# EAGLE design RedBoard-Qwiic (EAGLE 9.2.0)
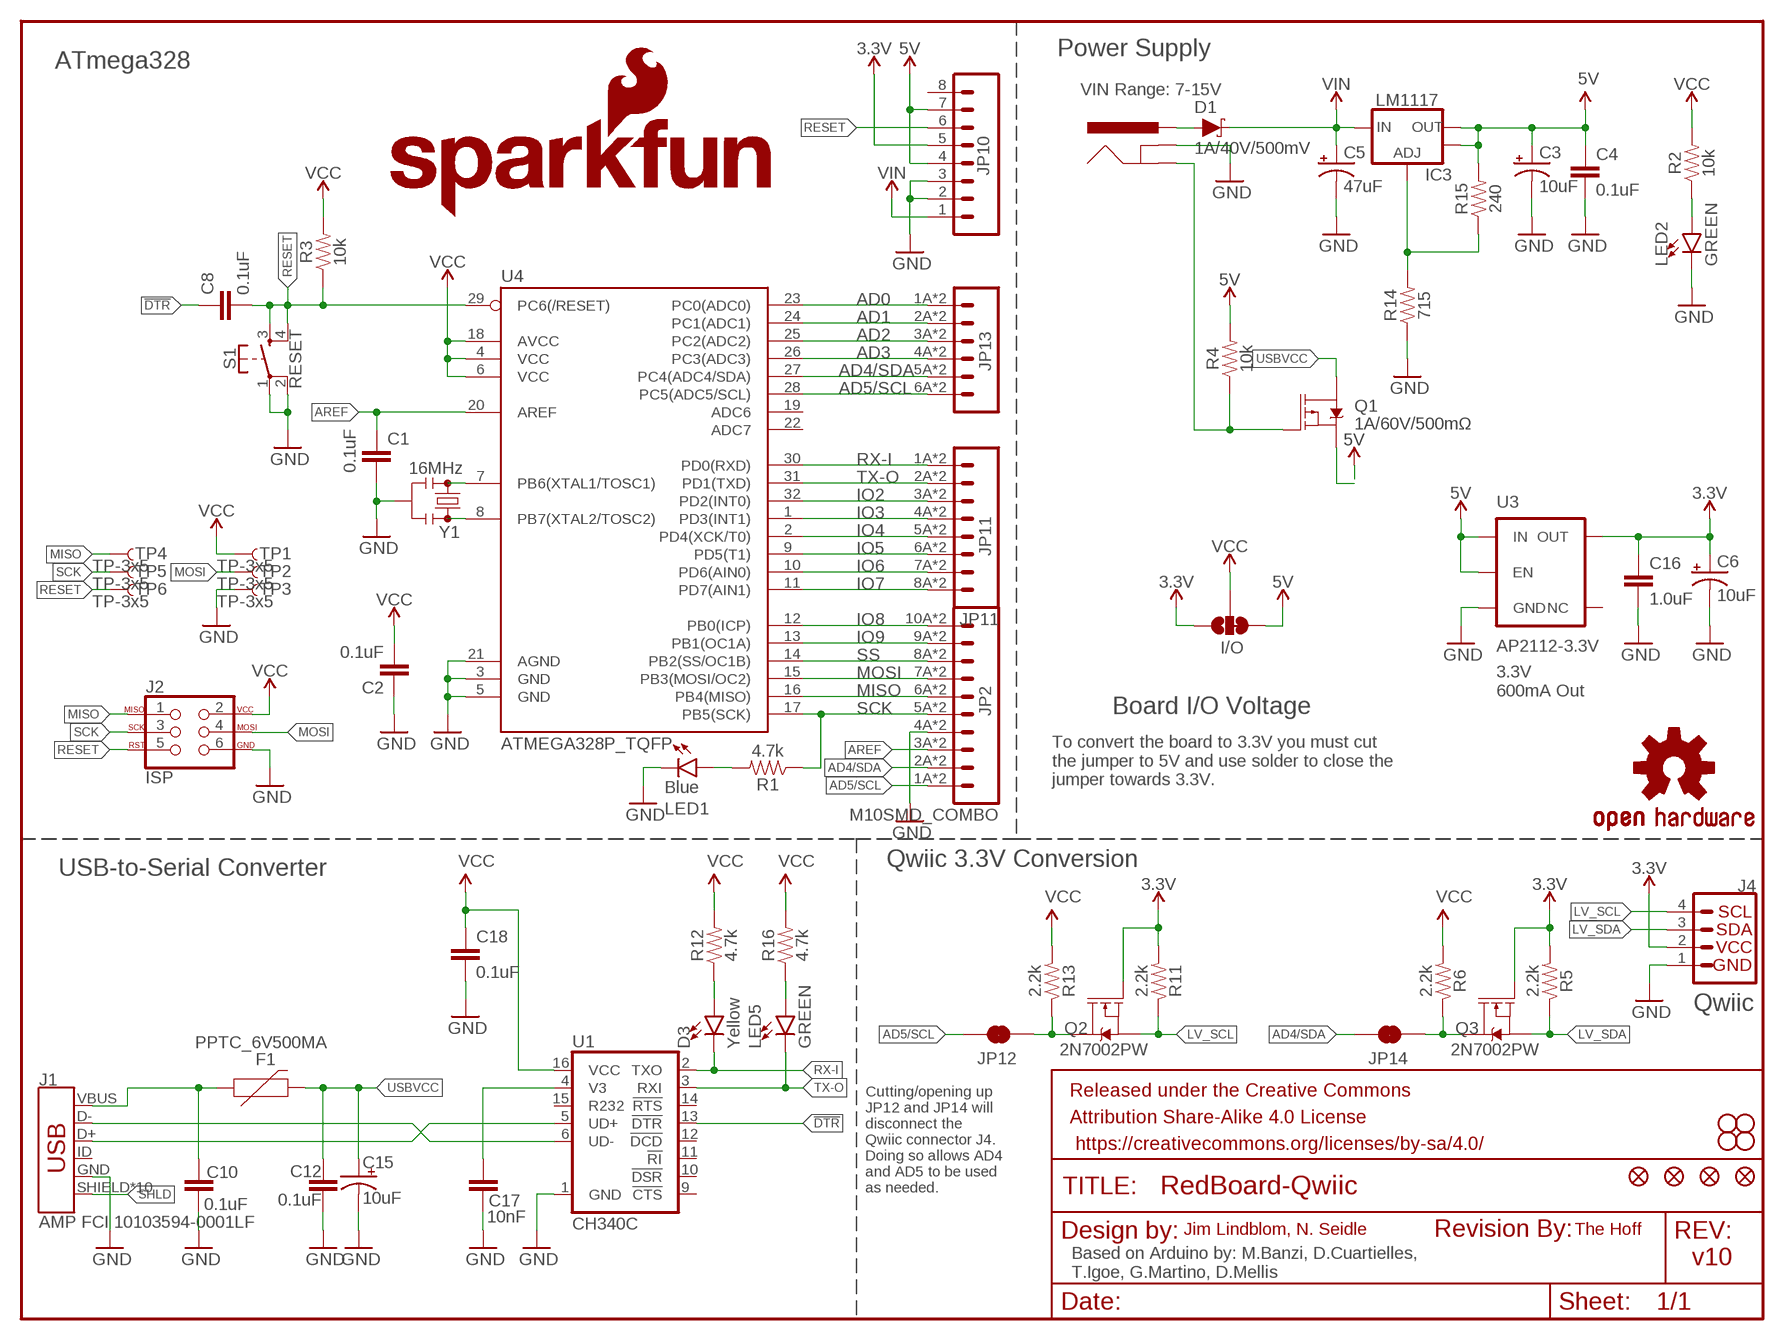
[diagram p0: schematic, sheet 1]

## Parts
C1  0.1uF  0.1UF-0603-25V-(+80/-20%)  [0603]
C2  0.1uF  0.1UF-0603-25V-(+80/-20%)  [0603]
C3  10uF  10UF-POLAR-EIA3216-16V-10%(TANT)  [EIA3216]
C4  0.1uF  0.1UF-0603-25V-(+80/-20%)  [0603]
C5  47uF  47UF-POLAR-PANASONIC_D-35V-20%  [PANASONIC_D]
C6  10uF  10UF-POLAR-EIA3216-16V-10%(TANT)  [EIA3216]
C8  0.1uF  0.1UF-0603-25V-(+80/-20%)  [0603]
C10  0.1uF  0.1UF-0603-25V-(+80/-20%)  [0603]
C12  0.1uF  0.1UF-0603-25V-(+80/-20%)  [0603]
C15  10uF  10UF-POLAR-EIA3216-16V-10%(TANT)  [EIA3216]
C16  1.0uF  1.0UF-16V-10%(0603)  [0603-CAP]
C17  10nF  10NF/10000PF-50V-10%(0603)  [0603-CAP]
C18  0.1uF  0.1UF-0603-25V-(+80/-20%)  [0603]
D1  1A/40V/500mV  DIODE-SCHOTTKY-SS14  [SMA-DIODE]
D3  Yellow  LED-YELLOW_HIDDENSILK  [LED-1206-HIDDENSILK]
F1  PPTC_6V500MA  [0805]
FRAME2  FRAME-LETTER  [CREATIVE_COMMONS]
I/O  JUMPER-SMT_3_1-NC_TRACE_SILK  [SMT-JUMPER_3_1-NC_TRACE_SILK]
IC3  LM1117  V_REG_LM1117ALT1  [SOT223-ALT1]
J1  AMP FCI 10103594-0001LF  USB_MICRO-B_HALF_PTH_MILL  [USB-MICROB-PTH-MILL]
J2  ISP  AVR_SPI_PROG_3X2SMD  [2X3_SMT_POSTS]
J3  POWER_JACKSUPER_BOMB_DIGITY  [POWER_JACK_SMD_OVERPASTE_SUPER_BOMB_DIGITY]
J4  QWIIC_CONNECTORJS-1MM  [1X04_1MM_RA]
JP1  SFE_LOGO_NAME.1_INCH  [SFE_LOGO_NAME_.1]
JP2  M10SMD_COMBO  [1X10_SMD_COMBINED]
JP3  STAND-OFF  [STAND-OFF]
JP4  STAND-OFF  [STAND-OFF]
JP5  STAND-OFF  [STAND-OFF]
JP6  STAND-OFF  [STAND-OFF]
JP7  SFE_LOGO_FLAME.1_INCH  [SFE_LOGO_FLAME_.1]
JP8  FIDUCIAL1X2  [FIDUCIAL-1X2]
JP9  FIDUCIAL1X2  [FIDUCIAL-1X2]
JP10  CONN_08SMD-COMBO-FEMALE  [1X08_SMD_COMBINED]
JP11  JP11  M08SMD-COMBO  [1X08_SMD_COMBINED@1]
JP12  JUMPER-SMT_2_NC_TRACE_SILK  [SMT-JUMPER_2_NC_TRACE_SILK]
JP13  M06SMD-STRAIGHT-COMBO  [1X06_SMD_STRAIGHT_COMBO]
JP14  JUMPER-SMT_2_NC_TRACE_SILK  [SMT-JUMPER_2_NC_TRACE_SILK]
JP15  FIDUCIAL1X2  [FIDUCIAL-1X2]
JP16  FIDUCIAL1X2  [FIDUCIAL-1X2]
LED1  Blue  LED-BLUE_HIDDENSILK  [LED-1206-HIDDENSILK]
LED2  GREEN  LED-GREEN_HIDDENSILK  [LED-1206-HIDDENSILK]
LED5  GREEN  LED-GREEN_HIDDENSILK  [LED-1206-HIDDENSILK]
LOGO1  REVISION  [REVISION]
Q1  1A/60V/500mΩ  MOSFET-PCH-ZXMP6A13F  [SOT23-3]
Q2  2N7002PW  MOSFET-NCH-2N7002PW  [SOT323]
Q3  2N7002PW  MOSFET-NCH-2N7002PW  [SOT323]
R1  4.7k  4.7KOHM-0603-1/10W-1%  [0603]
R2  10k  10KOHM-0603-1/10W-1%  [0603]
R3  10k  10KOHM-0603-1/10W-1%  [0603]
R4  10k  10KOHM-0603-1/10W-1%  [0603]
R5  2.2k  2.2KOHM-0603-1/10W-1%  [0603]
R6  2.2k  2.2KOHM-0603-1/10W-1%  [0603]
R11  2.2k  2.2KOHM-0603-1/10W-1%  [0603]
R12  4.7k  4.7KOHM-0603-1/10W-1%  [0603]
R13  2.2k  2.2KOHM-0603-1/10W-1%  [0603]
R14  715  715OHM-0603-1/10W-1%  [0603]
R15  240  240OHM-0603-1/10W-1%  [0603]
R16  4.7k  4.7KOHM-0603-1/10W-1%  [0603]
S1  RESET  MOMENTARY-SWITCH-SPST-2-SMD-5.2MM-TALL  [TACTILE_SWITCH_SMD_5.2MM]
TP1  TP-3x5  TEST-POINT3X5  [PAD.03X.05]
TP2  TP-3x5  TEST-POINT3X5  [PAD.03X.05]
TP3  TP-3x5  TEST-POINT3X5  [PAD.03X.05]
TP4  TP-3x5  TEST-POINT3X5  [PAD.03X.05]
TP5  TP-3x5  TEST-POINT3X5  [PAD.03X.05]
TP6  TP-3x5  TEST-POINT3X5  [PAD.03X.05]
U1  CH340C  [SO016]
U3  AP2112-3.3V  V_REG_AP2112K-3.3V  [SOT23-5]
U4  ATMEGA328P_TQFP  [TQFP32-08]
U$16  OSHW-LOGOS  [OSHW-LOGO-S]
Y1  16MHz  RESONATOR-16MHZSMD_3.2X1.3  [RESONATOR-SMD-3.2X1.3]

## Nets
3.3V: C6.+ C16.1 I/O.1 J4.2 JP10.5 Q2.1(G) Q3.1(G) R5.2 R11.2 U3.5(OUT)
5V: C3.+ C4.1 I/O.3 IC3.2(OUT) IC3.4(OUT) JP10.4 JP10.7 Q1.2(S) R4.2 R15.2 U3.1(IN) U3.3(EN)
!DTR: C8.1 U1.13(!DTR)
AD0: JP13.1A JP13.1B U4.23(PC0(ADC0))
AD1: JP13.2A JP13.2B U4.24(PC1(ADC1))
AD2: JP13.3A JP13.3B U4.25(PC2(ADC2))
AD3: JP13.4A JP13.4B U4.26(PC3(ADC3))
AD4/SDA: JP2.2A JP2.2B JP13.5A JP13.5B JP14.2 U4.27(PC4(ADC4/SDA))
AD5/SCL: JP2.1A JP2.1B JP12.2 JP13.6A JP13.6B U4.28(PC5(ADC5/SCL))
AREF: C1.1 JP2.3A JP2.3B U4.20(AREF)
GND: C1.2 C2.1 C3.- C4.2 C5.- C6.- C10.2 C12.2 C15.- C16.2 C17.2 C18.2 J1.GND J2.6 J3.GND(GNDBREAK) J4.1 JP2.4A JP2.4B JP10.2 JP10.3 LED1.C LED2.C R14.1 S1.1 S1.2 TP3.P$1 U1.1(GND) U3.2(GND) U4.3(GND) U4.5(GND) U4.21(AGND) Y1.2
INSERT: J3.P$4(GND) Q1.1(G) R4.1
IO2: JP11.3A JP11.3B U4.32(PD2(INT0))
IO3: JP11.4A JP11.4B U4.1(PD3(INT1))
IO4: JP11.5A JP11.5B U4.2(PD4(XCK/T0))
IO5: JP11.6A JP11.6B U4.9(PD5(T1))
IO6: JP11.7A JP11.7B U4.10(PD6(AIN0))
IO7: JP11.8A JP11.8B U4.11(PD7(AIN1))
IO8: JP2.10A JP2.10B U4.12(PB0(ICP))
IO9: JP2.9A JP2.9B U4.13(PB1(OC1A))
LV_SCL: J4.4 Q2.2(S) R11.1
LV_SDA: J4.3 Q3.2(S) R5.1
MISO: J2.1 JP2.6A JP2.6B TP4.P$1 U4.16(PB4(MISO))
MOSI: J2.4 JP2.7A JP2.7B TP2.P$1 U4.15(PB3(MOSI/OC2))
N$1: LED1.A R1.2
N$2: LED2.A R2.1
N$3: U4.7(PB6(XTAL1/TOSC1)) Y1.1
N$4: U4.8(PB7(XTAL2/TOSC2)) Y1.3
N$5: LED5.A R16.1
N$6: C17.1 U1.4(V3)
N$7: JP12.1 Q2.3(D) R13.1
N$8: JP14.1 Q3.3(D) R6.1
N$9: D3.A R12.1
N$13: J1.D- U1.6(UD-)
N$14: J1.D+ U1.5(UD+)
N$15: IC3.1(ADJ) R14.2 R15.1
PWRIN: D1.A J3.VIN0(PWR)
RESET: C8.2 J2.5 JP10.6 R3.1 S1.3 S1.4 TP6.P$1 U4.29(PC6(/RESET))
RX-I: D3.C JP11.1A JP11.1B U1.2(TXO) U4.30(PD0(RXD))
SCK: J2.3 JP2.5A JP2.5B R1.1 TP5.P$1 U4.17(PB5(SCK))
SHLD: J1.SHIELD J1.SHIELD2(SHIELD) J1.SHIELD3(SHIELD) J1.SHIELD4(SHIELD) J1.SHIELD5(SHIELD) J1.SHIELD6(SHIELD) J1.SHIELD7(SHIELD) J1.SHIELD8(SHIELD) J1.SHIELD9(SHIELD) J1.SHIELD10(SHIELD)
SS: JP2.8A JP2.8B U4.14(PB2(SS/OC1B))
TX-O: JP11.2A JP11.2B LED5.C U1.3(RXI) U4.31(PD1(TXD))
USBVCC: C12.1 C15.+ F1.2 Q1.3(D)
VCC: C2.2 C18.1 I/O.2 J2.2 R2.2 R3.2 R6.2 R12.2 R13.2 R16.2 TP1.P$1 U1.16(VCC) U4.4(VCC) U4.6(VCC) U4.18(AVCC)
VIN: C5.+ D1.C IC3.3(IN) JP10.1
VUSB: C10.1 F1.1 J1.VBUS
Unconnected: J1.ID JP10.8 U1.9(!CTS) U1.10(!DSR) U1.11(!RI) U1.12(!DCD) U1.14(!RTS) U1.15(R232) U3.4(NC) U4.19(ADC6) U4.22(ADC7)

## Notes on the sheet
- Power Supply
- ATmega328
- VIN Range: 7-15V
- 3.3V
  600mA Out
- Board I/O Voltage
- To convert the board to 3.3V you must cut
  the jumper to 5V and use solder to close the
  jumper towards 3.3V.
- Qwiic 3.3V Conversion
- USB-to-Serial Converter
- Qwiic
- Cutting/opening up
  JP12 and JP14 will 
  disconnect the 
  Qwiic connector J4.  
  Doing so allows AD4 
  and AD5 to be used
  as needed.
- Jim Lindblom, N. Seidle | The Hoff
- v10
- Based on Arduino by: M.Banzi, D.Cuartielles, 
  T.Igoe, G.Martino, D.Mellis

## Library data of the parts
C1 C2 C4 C8 C10 C12 C18 = SparkFun-Capacitors:0.1UF: 0.1µF ceramic capacitors; PROD_ID: CAP-00810
C3 C6 C15 = SparkFun-Capacitors:10UF-POLAR: 10.0µF polarized capacitors; PROD_ID: CAP-00811
C5 = SparkFun-Capacitors:47UF-POLAR: 47µF polarized capacitors; PROD_ID: CAP-08478
C16 = SparkFun-Capacitors:1.0UF-16V-10%(0603): CAP-00868; PROD_ID: CAP-00868
C17 = SparkFun-Capacitors:10NF/10000PF-50V-10%(0603): CAP-00867; PROD_ID: CAP-00867
D1 = SparkFun-DiscreteSemi:DIODE-SCHOTTKY: Schottky diode; PROD_ID: DIO-08053
D3 = SparkFun-LED:LED-YELLOW: Yellow SMD LED; PROD_ID: DIO-09909
F1 = SparkFun-Fuses:PPTC: Resettable Fuse PPTC
FRAME2 = SparkFun-Aesthetics:FRAME-LETTER: Schematic Frame - Letter
I/O = SparkFun-Jumpers:JUMPER-SMT_3_1-NC_TRACE: Normally closed trace jumper (1 of 2 connections) This jumper has a trace between two pads so it's normally closed (NC). The other connection is normally open (NO). Use a razor knife to open the connection. For best results follow the IPC guidelines for cutting traces: Cutout at least 0.063 mm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
IC3 = Testing:V_REG_LM1117: Voltage Regulator LM1117 Standard adjustable voltage regulator but in SMD form. Spark Fun Electronics SKU : COM-00595; PROD_ID: VREG-08170
J1 = SparkFun-Connectors:USB_MICRO-B: USB Type Micro-B Connector Male/female and PTH/SMT variants SparkFun Products: SparkFun microB USB Breakout SparkFun USB microB Plug Breakout SparkFun ESP8266 Thing; PROD_ID: CONN-13711
J2 = SparkFun-Connectors:AVR_SPI_PROG_3X2: AVR ISP 6 Pin This is the reduced ISP connector for AVR programming. Common on Arduino. This footprint will take up less PCB space and can be used with a 10-pin to 6-pin adapter such as SKU: BOB-08508 **Special note about "TEST_POINT" package. The stop mask is on the top side, so if you want your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; PROD_ID: CONN-11415
J3 = Testing:POWER_JACK: Power Jack This is the standard 5.5mm barrel jack for power. The PTH is the most common, proven, reliable, footprint. All others are experimental. The Slot footprint only works if the mill layer is transmitted to the PCB fab house so be warned. Spark Fun Electronics SKU : PRT-00119. Mating wall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; PROD_ID: CONN-08106
J4 = SparkFun-Connectors:QWIIC_CONNECTOR: SparkFun I2C Standard Qwiic Connector An SMD 1mm pitch JST connector makes it easy and quick (get it? Qwiic?) to connect I2C devices to each other. The Qwiic system enables fast and solderless connection between popular platforms and various sensors and actuators. We carry 200mm, 100mm, 50mm, and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; PROD_ID: CONN-13694
JP1 = SparkFun-Aesthetics:SFE_LOGO_NAME: SFE Logo, name only
JP2 = SparkFun-Connectors:M10: Header 10 Standard 10-pin 0.1" header. Use with straight break away headers (SKU : PRT-00116), right angle break away headers (PRT-00553), swiss pins (PRT-00743), machine pins (PRT-00117), and female headers (PRT-00115).; PROD_ID: CONN-11219
JP3-JP6 = SparkFun:STAND-OFF: Stand Off
JP7 = SparkFun-Aesthetics:SFE_LOGO_FLAME: SFE Logo, flame only
JP8 JP9 JP15 JP16 = SparkFun:FIDUCIAL: Fiducial Alignment Points
JP10 = SparkFun-Connectors:CONN_08: Multi connection point. Often used as Generic Header-pin footprint for 0.1 inch spaced/style header connections On any of the 0.1 inch spaced packages, you can populate with these: Break Away Headers - Straight (PRT-00116) Break Away Male Headers - Right Angle (PRT-00553) Female Headers (PRT-00115)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; PROD_ID: CONN-10204; SF_ID: PRT-11543
JP11 = SparkFun-Connectors:M08: Header 8 Standard 8-pin 0.1" header. Use with straight break away headers (SKU : PRT-00116), right angle break away headers (PRT-00553), swiss pins (PRT-00743), machine pins (PRT-00117), and female headers (PRT-00115).; PROD_ID: CONN-10204
JP12 JP14 = SparkFun-Jumpers:JUMPER-SMT_2_NC_TRACE: Normally closed trace jumper
JP13 = SparkFun-Connectors:M06: Header 6 Standard 6-pin 0.1" header. Use with straight break away headers (SKU : PRT-00116), right angle break away headers (PRT-00553), swiss pins (PRT-00743), machine pins (PRT-00117), and female headers (PRT-00115). Molex polarized connector foot print use with SKU : PRT-08094 with associated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; PROD_ID: CONN-10203
LED1 = SparkFun-LED:LED-BLUE: Blue SMD LED; PROD_ID: DIO-09911
LED2 = SparkFun-LED:LED-GREEN: Green SMD LED; PROD_ID: DIO-09910
LED5 = SparkFun-LED:LED-GREEN: Green SMD LED; PROD_ID: DIO-00862
LOGO1 = SparkFun-Aesthetics:REVISION: "Revision By" Text
Q1 = SparkFun-DiscreteSemi:MOSFET-PCH: P-channel MOSFETs Voltage controlled devices that allow control of high current outputs.; PROD_ID: TRANS-08285
Q2 Q3 = SparkFun-DiscreteSemi:MOSFET-NCH: N-channel MOSFETs Voltage controlled devices that allow control of high current outputs.; PROD_ID: TRANS-11151; VALUE: 310mA/60V/1.6Ω
R1 R12 R16 = SparkFun-Resistors:4.7KOHM: 4.7kΩ resistor; PROD_ID: RES-07857
R2-R4 = SparkFun-Resistors:10KOHM: 10kΩ resistor; PROD_ID: RES-00824
R5 R6 R11 R13 = SparkFun-Resistors:2.2KOHM: 2.2kΩ resistor; PROD_ID: RES-08272
R14 = SparkFun-Resistors:715OHM: 715Ω resistor; PROD_ID: RES-07850
R15 = SparkFun-Resistors:240OHM: 240Ω resistor; PROD_ID: RES-07849
S1 = SparkFun-Switches:MOMENTARY-SWITCH-SPST-2: Momentary Switch (Pushbutton) - SPST - Two Circuits Normally-open (NO) SPST momentary switches (buttons, pushbuttons). Schematic symbol includes two switch circuits. Variants SMD-4.6MMX2.8MM - 4.60mm x 2.80mm Tactile Momentary Button Switch - Used on SparkFun SAMD21 Mini Breakout SMD-5.2MM - Mini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; PROD_ID: SWCH-14139
TP1-TP4 TP6 = SparkFun-Connectors:TEST-POINT: Bare copper test points for troubleshooting or ICT
TP5 = SparkFun-Passives:TEST-POINT: Bare copper test points for troubleshooting or ICT
U1 = SparkFun-IC-Comms:CH340C; PROD_ID: IC-14038
U3 = SparkFun-PowerIC:V_REG_AP2112: AP2112 - 600mA CMOS LDO Regulator w/ Enable The AP2112 is CMOS process low dropout linear regulator with enable function, the regulator delivers a guaranteed 600mA (min.) continuous load current. Features Output Voltage Accuracy: ±1.5% Output Current: 600mA (Min.) Foldback Short Current Protection: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; PROD_ID: VREG-12457; VALUE: 3.3V
U4 = SparkFun-IC-Microcontroller:ATMEGA328P_TQFP; PROD_ID: IC-09069
U$16 = SparkFun-Aesthetics:OSHW-LOGO: Open Source Hardware Logo
Y1 = SparkFun-Clocks:RESONATOR-16MHZ: 16MHz Resonator Digikey Example Frequency: 16MHz Frequency Stability: &plusmn;0.3% Frequency Tolerance: &plusmn;0.5% Capacitance: 15pF; PROD_ID: XTAL-08900

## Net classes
1 power: width 0.178 mm

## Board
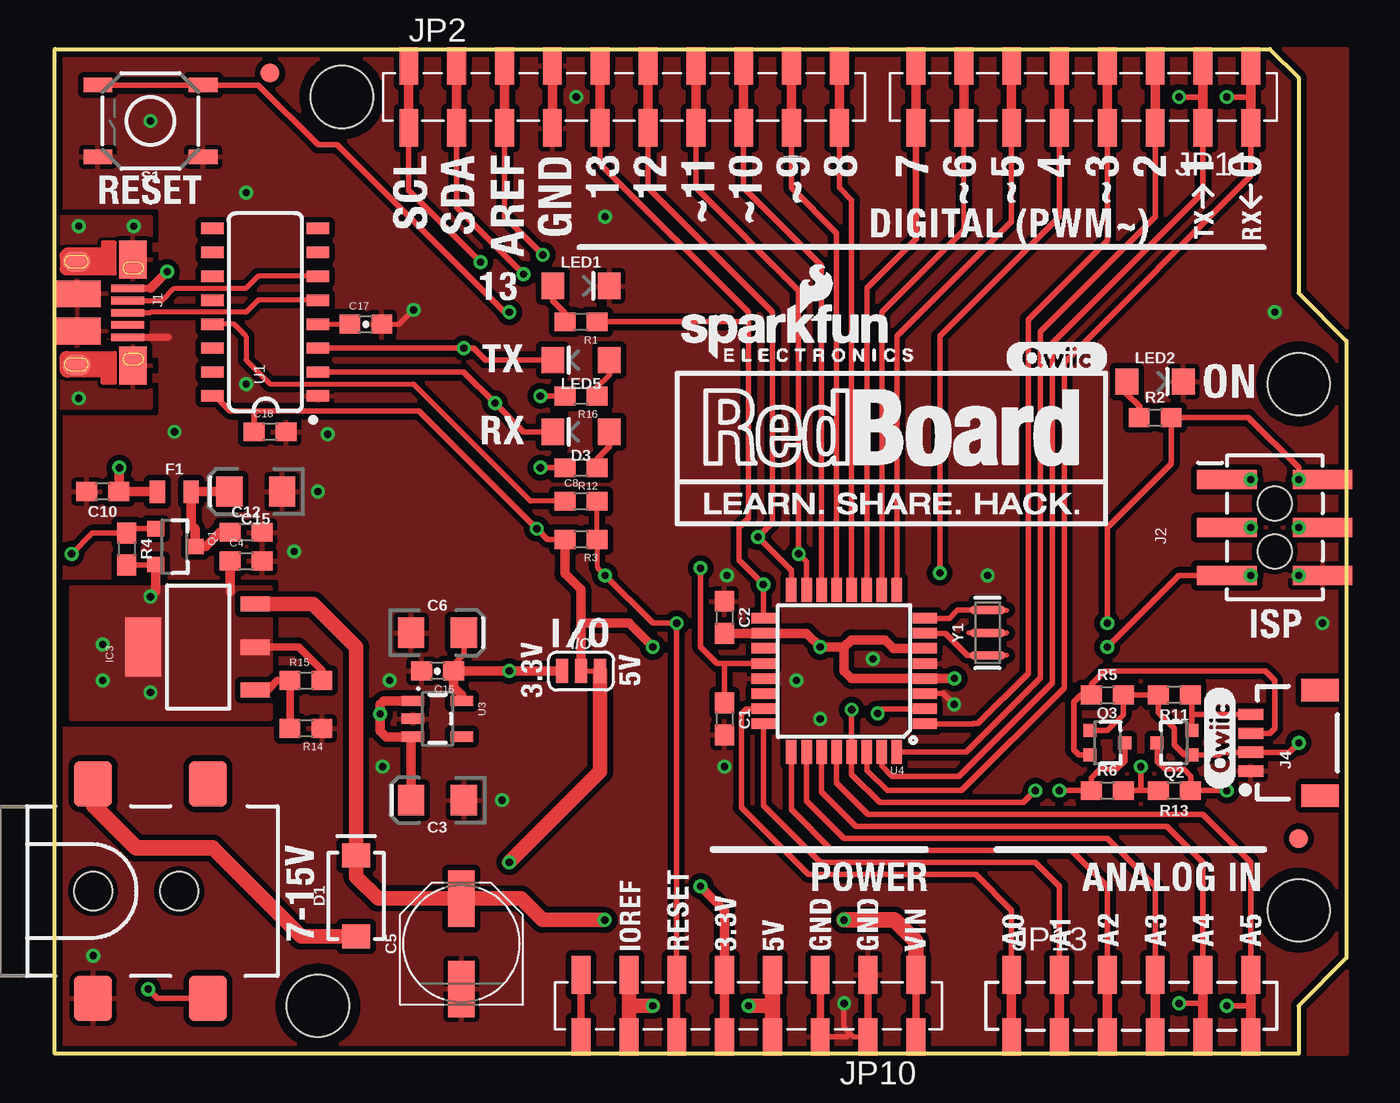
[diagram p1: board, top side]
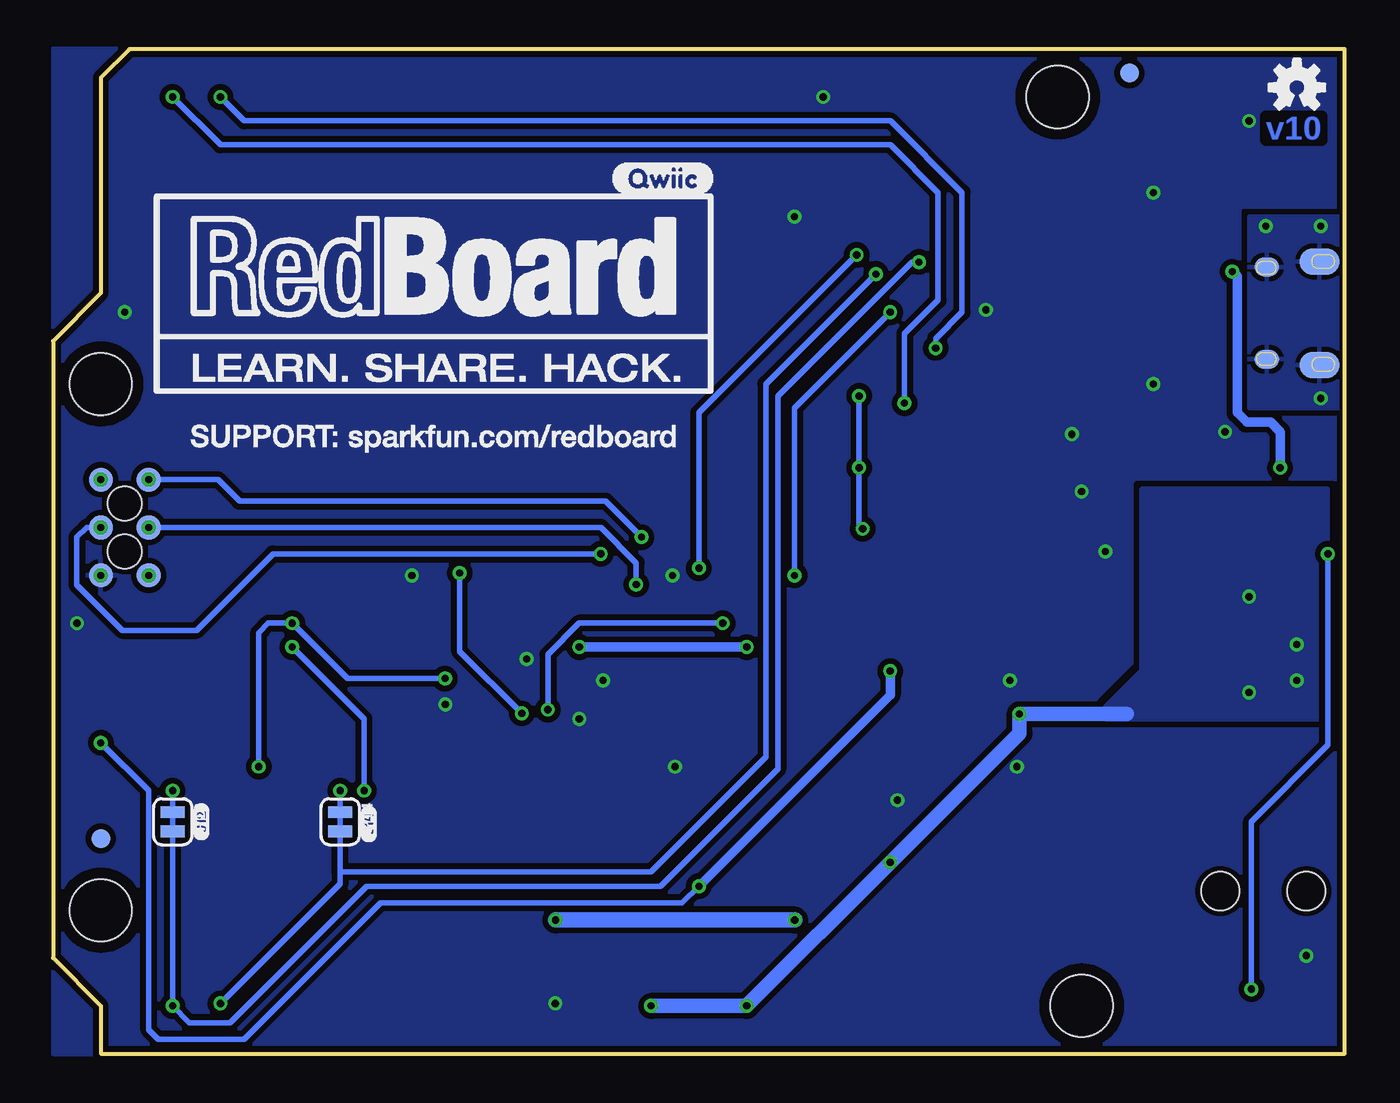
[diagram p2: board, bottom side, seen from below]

Size 68.58 x 53.34 mm. Coordinates in mm from the lower left corner, seen from the top.
Outline: 0,53.34 64.52,53.34 66.04,51.82 66.04,40.39 68.58,37.85 68.58,5.08 66.04,2.54 66.04,0 0,0 0,53.34
Copper layers (1*16): Top 0.035mm / dielectric 1.5mm / Bottom 0.035mm
Design rules "SparkFun-2-layer-TIGHT": minimum track width 7mil, minimum drill 15mil, track to track 7mil, track to pad 7mil, pad to pad 7mil, via to via 7mil, smd to smd 7mil, copper to edge 7mil, drill to drill 7mil, minimum pad ring 7mil, minimum via ring 7mil, stop-mask expansion 4mil, vias tented up to drill 25mil, thermal gap 10mil
vRestrict: area 0.6,22.4 to 2,30.6; area 5.7,23.1 to 7.4,30.6; area 47.9,10.8 to 48.5,11.3; area 50.4,10.7 to 50.9,11.6; area 11.3,29.3 to 12.7,31.6; area 0.3,13 to 9.4,25

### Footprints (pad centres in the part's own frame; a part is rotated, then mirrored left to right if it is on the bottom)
0603 = smd 1.1 x 1: 1 -0.85,0; 2 0.85,0
EIA3216 = smd 1.4 x 1.6: + 1.4,0; - -1.4,0
PANASONIC_D = smd 3 x 1.4: + 2.4,0; - -2.4,0
0603-CAP = smd 1.1 x 1: 1 -0.85,0; 2 0.85,0
SMA-DIODE = smd 1.27 x 1.47: A -2.15,0; C 2.15,0
LED-1206-HIDDENSILK = smd 1.2 x 1.4: A -1.5,0; C 1.5,0
0805 = smd 0.8 x 1.2: 1 -0.9,0; 2 0.9,0
SMT-JUMPER_3_1-NC_TRACE_SILK = smd 0.635 x 1.27: 1 -1.016,0; 2 0,0; 3 1.016,0
SOT223-ALT1 = smd 0.813 x 1.524: 1 -2.271,-3.02; 2 0,-3.02; 3 2.288,-3.02 | smd 3.124 x 1.905: 4 0,2.921
USB-MICROB-PTH-MILL = smd 0.4 x 1.75: D+ 0.031,1.331; D- -0.619,1.331; GND 1.331,1.331; ID 0.681,1.331; VBUS -1.269,1.331 | smd 2 x 1.46: SHIELD -2.794,1.606; SHIELD2 2.831,1.606 | smd 1.425 x 2.5: SHIELD3 -0.979,-1.349; SHIELD4 0.996,-1.352 | smd 1.4 x 2.1 bottom: SHIELD5 -2.7,-1.2; SHIELD7 2.8,-1.2 | smd 1.1 x 1.5: SHIELD6 2.8,-1.4; SHIELD8 -2.7,-1.4 | smd 1 x 1.3 bottom: SHIELD9 -2.4,1.6; SHIELD10 2.5,1.6
2X3_SMT_POSTS = smd 1 x 3.17: 1 -2.54,-2.54; 2 -2.54,2.54; 3 0,-2.54; 4 0,2.54; 5 2.54,-2.54; 6 2.54,2.54 | hole 1.8: -1.27,0; 1.27,0
POWER_JACK_SMD_OVERPASTE_SUPER_BOMB_DIGITY = smd 2 x 2.4: GND 0,-5.7; P$4 6.1,-5.7; VIN0 0,5.7; VIN1 6.1,5.7 | hole 2.032: 0,0; 4.572,0
1X04_1MM_RA = smd 0.6 x 1.35: 1 -1.5,0; 2 -0.5,0; 3 0.5,0; 4 1.5,0 | smd 1.2 x 2: NC1 2.8,-3.675; NC2 -2.8,-3.675
1X10_SMD_COMBINED = smd 1 x 2: 1A 0,1.65; 1B 0,-1.65; 2A 2.54,1.65; 2B 2.54,-1.65; 3A 5.08,1.65; 3B 5.08,-1.65; 4A 7.62,1.65; 4B 7.62,-1.65; 5A 10.16,1.65; 5B 10.16,-1.65; 6A 12.7,1.65; 6B 12.7,-1.65; 7A 15.24,1.65; 7B 15.24,-1.65; 8A 17.78,1.65; 8B 17.78,-1.65; 9A 20.32,1.65; 9B 20.32,-1.65; 10A 22.86,1.65; 10B 22.86,-1.65
STAND-OFF = hole 3.302: 0,0
FIDUCIAL-1X2 = smd 1 x 1: 1 0,0
1X08_SMD_COMBINED = smd 1 x 2: 1 0,1.65; 1@2 0,-1.65; 2 2.54,-1.65; 2@2 2.54,1.65; 3 5.08,1.65; 3@2 5.08,-1.65; 4 7.62,-1.65; 4@2 7.62,1.65; 5 10.16,1.65; 5@2 10.16,-1.65; 6 12.7,-1.65; 6@2 12.7,1.65; 7 15.24,1.65; 7@2 15.24,-1.65; 8 17.78,-1.65; 8@2 17.78,1.65
1X08_SMD_COMBINED@1 = smd 1 x 2: 1A 0,1.65; 1B 0,-1.65; 2A 2.54,-1.65; 2B 2.54,1.65; 3A 5.08,1.65; 3B 5.08,-1.65; 4A 7.62,-1.65; 4B 7.62,1.65; 5A 10.16,1.65; 5B 10.16,-1.65; 6A 12.7,-1.65; 6B 12.7,1.65; 7A 15.24,1.65; 7B 15.24,-1.65; 8A 17.78,-1.65; 8B 17.78,1.65
SMT-JUMPER_2_NC_TRACE_SILK = smd 0.635 x 1.27: 1 -0.508,0; 2 0.508,0
1X06_SMD_STRAIGHT_COMBO = smd 1 x 2: 1A 0,-1.65; 1B 0,1.65; 2A 2.54,1.65; 2B 2.54,-1.65; 3A 5.08,-1.65; 3B 5.08,1.65; 4A 7.62,1.65; 4B 7.62,-1.65; 5A 10.16,-1.65; 5B 10.16,1.65; 6A 12.7,1.65; 6B 12.7,-1.65
SOT23-3 = smd 0.8 x 0.9: 1 -0.95,-1; 2 0.95,-1; 3 0,1.1
SOT323 = smd 0.7 x 0.7: 1 -0.65,-0.925; 2 0.65,-0.925; 3 0,0.925
TACTILE_SWITCH_SMD_5.2MM = smd 1.524 x 0.762: 1 -2.794,1.905; 2 2.794,1.905; 3 -2.794,-1.905; 4 2.794,-1.905
PAD.03X.05 = smd 1.27 x 1.27: P$1 0,0
SO016 = smd 0.6 x 1.2: 1 -4.445,-2.8; 2 -3.175,-2.8; 3 -1.905,-2.8; 4 -0.635,-2.8; 5 0.635,-2.8; 6 1.905,-2.8; 7 3.175,-2.8; 8 4.445,-2.8; 9 4.445,2.8; 10 3.175,2.8; 11 1.905,2.8; 12 0.635,2.8; 13 -0.635,2.8; 14 -1.905,2.8; 15 -3.175,2.8; 16 -4.445,2.8
SOT23-5 = smd 0.55 x 1.2: 1 -0.95,-1.3; 2 0,-1.3; 3 0.95,-1.3; 4 0.95,1.3; 5 -0.95,1.3
TQFP32-08 = smd 1.27 x 0.559: 1 -4.293,2.8; 2 -4.293,2; 3 -4.293,1.2; 4 -4.293,0.4; 5 -4.293,-0.4; 6 -4.293,-1.2; 7 -4.293,-2; 8 -4.293,-2.8; 17 4.293,-2.8; 18 4.293,-2; 19 4.293,-1.2; 20 4.293,-0.4; 21 4.293,0.4; 22 4.293,1.2; 23 4.293,2; 24 4.293,2.8 | smd 0.559 x 1.27: 9 -2.8,-4.293; 10 -2,-4.293; 11 -1.2,-4.293; 12 -0.4,-4.293; 13 0.4,-4.293; 14 1.2,-4.293; 15 2,-4.293; 16 2.8,-4.293; 25 2.8,4.293; 26 2,4.293; 27 1.2,4.293; 28 0.4,4.293; 29 -0.4,4.293; 30 -1.2,4.293; 31 -2,4.293; 32 -2.8,4.293
RESONATOR-SMD-3.2X1.3 = smd 0.45 x 1.905: 1 -1.2,0; 2 0,0; 3 1.2,0

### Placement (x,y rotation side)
C1  35.56,17.78 270 top
C2  35.56,23.17 270 top
C3  20.32,13.46 180 top
C4  10.16,26.16 0 top
C5  21.59,5.84 90 top
C6  20.32,22.35 0 top
C8  27.94,29.34 0 top
C10  2.54,29.84 180 top
C12  10.16,27.69 0 top
C15  10.67,29.84 180 top
C16  20.32,20.32 180 top
C17  16.51,38.73 0 top
C18  11.43,33.02 0 top
D1  16,8.38 90 top
D3  27.94,33.02 180 top
F1  6.35,29.84 0 top
FRAME2  not placed on the board
I/O  27.94,20.32 0 top
IC3  7.62,21.59 90 top
J1  2.54,39.37 270 top
J2  64.77,27.94 270 top
J3  2.03,8.64 0 top
J4  63.5,16.51 90 top
JP1  32.79,36.45 0 top
JP2  18.8,50.8 0 top
JP3  13.97,2.54 0 top
JP4  66.04,7.62 0 top
JP5  66.04,35.56 0 top
JP6  15.24,50.8 0 top
JP7  39.27,38.99 0 top
JP8  66.04,11.43 0 top
JP9  11.43,52.07 0 top
JP10  45.72,2.54 180 top
JP11  63.5,50.8 180 top
JP12  62.23,12.32 270 bottom
JP13  50.8,2.54 0 top
JP14  53.34,12.32 270 bottom
JP15  11.43,52.07 0 bottom
JP16  66.04,11.43 0 bottom
LED1  27.94,40.77 0 top
LED2  58.42,35.69 0 top
LED5  27.94,36.83 180 top
LOGO1  not placed on the board
Q1  6.35,26.92 270 top
Q2  59.44,16.51 90 top
Q3  55.88,16.51 270 top
R1  27.94,38.86 180 top
R2  58.42,33.78 0 top
R3  27.94,27.3 180 top
R4  3.81,26.8 270 top
R5  55.88,19.05 0 top
R6  55.88,13.97 0 top
R11  59.44,19.05 180 top
R12  27.94,31.11 180 top
R13  59.44,13.97 180 top
R14  13.34,17.27 180 top
R15  13.34,19.81 0 top
R16  27.94,34.92 180 top
S1  5.08,49.53 180 top
TP1  66.04,30.48 0 bottom
TP2  66.04,27.94 0 bottom
TP3  66.04,25.4 0 bottom
TP4  63.5,30.48 0 bottom
TP5  63.5,27.94 0 bottom
TP6  63.5,25.4 0 bottom
U1  11.18,39.37 90 top
U3  20.32,17.78 270 top
U4  41.91,20.32 180 top
U$1  [(QWIIC)]  50.42,36.96 0 top
U$2  [(QWIIC)]  61.85,13.97 90 top
U$3  [(QWIIC)]  38.99,46.48 0 bottom
U$4  [J120]  60.71,11.3 90 bottom
U$9  [J140]  51.82,11.18 90 bottom
U$16  2.54,51.31 0 bottom
Y1  49.53,22.35 90 top

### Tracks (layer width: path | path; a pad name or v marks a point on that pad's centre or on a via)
3.3V  (via drill 0.38)
  Top 0.254: 35.56,4.19 JP10.5
  Top 0.305: C6.+ 21.72,21.21 21.17,20.66 C16.1 | Q3.1 55.9,17.16 56.73,18 R5.2 R11.2 58.59,18.12 59.44,17.27 59.44,16.38 59.96,15.86 Q2.1 61.83,15.86 61.98,16.01 J4.2 65.54,16.01 v66.04,16.51
  Top 0.508: JP10.5 35.56,7.62 v34.29,8.89 | I/O.1 v24.13,20.32 C16.1 21.17,19.47 21.59,19.05 21.59,18.76 U3.5
  Bottom 0.305: v34.29,8.89 35.18,8 51.18,8 58.42,0.76 62.99,0.76 63.5,1.27 63.5,13.97 v66.04,16.51
  Bottom 0.508: v24.13,20.32 24.13,19.05 v34.29,8.89
5V  (via drill 0.38)
  Top 0.305: JP10.4 38.1,2.03 | R4.2 5.32,25.95 Q1.2
  Top 0.406: IC3.2 12.95,21.59 14.19,20.36 R15.2
  Top 0.508: C3.+ 18.92,16.73 U3.3 17.59,16.83 17.27,17.14 v17.27,18.03 17.27,18.54 17.46,18.73 U3.1 | Q1.2 5.35,24.54 v5.08,24.27 | C4.1 9.31,24.55
  Top 0.762: v36.83,2.54 37.85,2.54 38.1,2.79 | v31.75,2.54 30.48,2.54 | 30.48,2.54 JP10.7 | 30.48,4.19 30.48,2.54 | I/O.3 28.96,14.99 v24.13,10.16
  Top 0.813: JP10.4 38.1,2.79 38.1,2.03 38.1,0.89
  Bottom 0.762: v36.83,2.54 v31.75,2.54 v24.13,10.16 17.27,17.02 v17.27,18.03 11.56,18.03
  other vias: 2.54,21.73 5.08,19.19 2.54,19.82
  pour Bottom (isolate 0.305, no thermals): 0.89,29.97 10.79,29.97 10.79,20.32 12.7,18.41 12.7,17.78 0.89,17.78
  pour Top (isolate 0.305, no thermals): 0.89,17.78 0.89,24.77 11.43,24.77 11.43,17.78
!DTR
  Top 0.254: C8.1 25.27,29.34 19.05,35.56 11.43,35.56 10.16,36.83 10.16,38.1 9.53,38.73 U1.13
AD0
  Top 0.254: JP13.1B JP13.1A
  Top 0.305: JP13.1A 50.8,7.62 48.9,9.53 40.01,9.53 36.45,13.08 36.45,18.03 36.73,18.32 U4.23
AD1
  Top 0.254: JP13.2A JP13.2B
  Top 0.305: U4.24 37.62,13.18 40.64,10.16 52.07,10.16 53.34,8.89 JP13.2A
AD2
  Top 0.254: JP13.3B 55.88,1.27
  Top 0.305: U4.25 39.11,12.96 41.27,10.79 53.98,10.79 55.88,8.89 55.88,1.27 JP13.3A
AD3
  Top 0.254: JP13.4A JP13.4B
  Top 0.305: U4.26 39.91,13.43 41.91,11.43 55.88,11.43 58.42,8.89 JP13.4A
AD4/SDA  (via drill 0.38)
  Top 0.254: JP13.5B 60.96,2.67 | JP2.2A JP2.2B
  Top 0.305: U4.27 40.71,13.9 42.55,12.06 59.05,12.06 60.96,10.16 60.96,2.67 | 60.96,2.67 JP13.5A | JP2.2B 21.34,44.96 v24.89,41.4 | v59.69,2.67 60.96,2.67
  Bottom 0.305: 53.34,9.65 36.83,9.65 30.73,15.75 30.73,35.56 v24.89,41.4 | v59.69,2.67 53.34,9.02 53.34,9.65 | 53.34,9.65 JP14.2
AD5/SCL  (via drill 0.38)
  Top 0.254: 63.5,2.54 JP13.6B | JP2.1A JP2.1B
  Top 0.305: U4.28 41.51,14.37 43.18,12.7 60.2,12.7 60.96,12.7 63.5,10.16 JP13.6A 63.5,2.54 v62.23,2.54 | JP2.1B 18.8,45.85 v22.61,42.04
  Bottom 0.305: JP12.2 v62.23,2.54 61.34,1.65 59.18,1.65 51.94,8.89 36.32,8.89 30.1,15.11 30.1,34.92 22.99,42.04 v22.61,42.04
AREF  (via drill 0.38)
  Top 0.254: JP2.3A JP2.3B
  Top 0.305: 35.56,20.72 35.16,20.72 34.29,21.59 v34.29,25.78 | 35.56,20.72 U4.20 | C1.1 35.56,20.72 | JP2.3B 23.88,44.45 v25.91,42.42
  Bottom 0.305: v25.91,42.42 34.29,34.04 v34.29,25.78
GND  (via drill 0.38, 0.38 pad 0.51)
  Top 0.254: 43.18,0.89 42.42,0.89 42.23,1.08 41.91,1.4 v41.91,2.67 | C17.2 18.29,38.73 v19.05,39.5
  Top 0.305: U4.3 47.17,19.12 v47.75,18.54 | JP10.3 42.04,0.89 42.23,1.08
  Top 0.381: J1.GND 6.04,38.04
  other vias: 5.08,49.53 64.77,39.37 40.64,17.78 27.69,50.8 43.43,20.95 49.53,25.4 35.69,25.4 2.03,5.21 29.21,44.45 67.31,22.86 17.78,19.81 17.4,15.24 66.04,25.4 6.35,33.02 13.97,29.84 14.48,32.89 12.7,26.67 10.16,35.56 10.16,45.72 23.75,13.46 35.56,15.24 39.37,19.81
  pour Top (isolate 0.305, rank 2): 0,53.34 68.58,53.34 68.58,0 0,0
  pour Bottom (isolate 0.305, rank 2): 0,53.34 68.58,53.34 68.58,0 0,0
INSERT  (via drill 0.38)
  Top 0.305: J3.P$4 5.45,2.94 v4.95,3.43 | Q1.1 4.04,27.87 R4.1 1.99,27.65 v0.89,26.54
  Bottom 0.305: v4.95,3.43 4.95,12.32 0.89,16.38 v0.89,26.54
IO2
  Top 0.254: JP11.3B JP11.3A
  Top 0.305: JP11.3A 58.42,44.45 52.32,38.35 52.32,19.94 48.41,16.03 U4.32
IO3
  Top 0.254: JP11.4A 55.88,49.53 | JP11.4B 55.88,48.26
  Top 0.305: 55.88,49.53 55.88,48.26 55.88,43.18 51.69,38.99 51.69,20.19 49.02,17.53 48.77,17.53 48.76,17.52 U4.1
IO4  (via drill 0.38)
  Top 0.254: JP11.5B JP11.5A
  Top 0.305: v46.99,25.53 46.99,38.1 53.34,44.45 JP11.5A | U4.2 43.94,18.32 v43.69,18.07
  Bottom 0.305: v43.69,18.07 46.99,21.37 v46.99,25.53
IO5
  Top 0.254: JP11.6A JP11.6B
  Top 0.305: U4.9 44.71,38.1 50.8,44.19 JP11.6B
IO6
  Top 0.254: 48.26,43.72 JP11.7A JP11.7B
  Top 0.305: U4.10 43.91,39.37 48.26,43.72
IO7
  Top 0.254: JP11.8A 45.72,49.53 JP11.8B
  Top 0.305: U4.11 43.11,40.64 45.72,43.25
  Top 0.356: 45.72,49.53 45.72,43.25
IO8
  Top 0.254: JP2.10A JP2.10B
  Top 0.305: U4.12 42.31,45.32 41.66,45.97 JP2.10B
IO9
  Top 0.254: JP2.9A JP2.9B
  Top 0.305: U4.13 41.51,43.58 39.12,45.97 JP2.9B
LV_SCL
  Top 0.305: Q2.2 60.36,18.03 | 60.36,18.03 60.36,18.98 R11.1 | J4.4 60.38,18.01 60.36,18.03
LV_SDA
  Top 0.305: J4.3 64.51,17.01 64.77,17.27 64.77,19.81 64.26,20.32 55.75,20.32 55.03,19.6 R5.1 54.48,19.05 54.1,18.67 54.1,16.13 54.37,15.86 Q3.2
MISO  (via drill 0.38, 0.38 pad 0.51)
  Top 0.254: JP2.6A JP2.6B
  Top 0.305: U4.16 39.11,25.66 v37.34,27.43 38.1,28.19 38.1,39.37 31.5,45.97 JP2.6B | J2.1 TP4.P$1
  Bottom 0.305: v37.34,27.43 39.24,29.34 58.67,29.34 59.82,30.48 TP4.P$1
  other vias: 63.5,30.48
MOSI  (via drill 0.38, 0.38 pad 0.51)
  Top 0.254: JP2.7A JP2.7B
  Top 0.305: U4.15 39.91,26.13 v39.5,26.54 39.5,40.51 34.04,45.97 JP2.7B | J2.4 TP2.P$1
  Bottom 0.305: v39.5,26.54 56.9,26.54 60.96,22.48 64.9,22.48 67.31,24.89 67.31,27.43 66.8,27.94 TP2.P$1
  other vias: 66.04,27.94
N$1
  Top 0.305: R1.2 27.09,39.33 26.44,39.98 LED1.A
N$2
  Top 0.356: R2.1 57.57,34.38 56.92,35.03 LED2.A
N$3
  Top 0.305: U4.7 47.28,22.32 48.44,21.15 Y1.1
N$4
  Top 0.305: U4.8 47.5,23.12 47.94,23.55 Y1.3
N$5
  Top 0.305: R16.1 28.79,35.39 29.44,36.04 LED5.A
N$6
  Top 0.254: U1.4 C17.1
N$7  (via drill 0.38)
  Top 0.305: Q2.3 58.55,16.47 58.55,15.49 58.93,15.11 59.94,15.11 60.33,14.73 60.33,14.01 R13.1 v62.23,13.97
  Bottom 0.305: JP12.1 v62.23,13.97
N$8  (via drill 0.38)
  Top 0.305: v53.34,13.97 R6.1 55.03,14.64 55.5,15.11 56.39,15.11 56.8,15.53 Q3.3
  Bottom 0.305: JP14.1 v53.34,13.97
N$9
  Top 0.305: R12.1 28.79,31.58 29.44,32.23 D3.A
N$13
  Top 0.254: J1.D- 5.7,39.99 6.35,40.64 10.16,40.64 10.79,41.27 U1.6
N$14
  Top 0.254: J1.D+ 4.83,39.34 5.05,39.34 5.08,39.37 10.16,39.37 10.79,40.01 U1.5
N$15
  Top 0.406: IC3.1 11.32,19.32 11.81,19.81 R15.1 R14.2
PWRIN
  Top 0.762: 8.38,10.92 13.07,6.23 D1.A
  Top 0.813: 8.38,10.92 4.32,10.92 2.03,13.21 J3.VIN0
RESET  (via drill 0.38, 0.38 pad 0.51)
  Top 0.254: C8.2 R3.1 28.79,25.82 v29.21,25.4
  Top 0.305: v42.31,18.27 U4.29 42.31,14.84 43.81,13.34 51.44,13.34 v52.07,13.97 | 33.02,0.89 JP10.6 v33.02,22.86 31.75,22.86 v29.21,25.4 | TP6.P$1 J2.5 59.69,25.4 v55.88,21.59 | S1.4 S1.3 10.79,51.44 13.97,48.26 14.99,48.26 23.88,39.37 v24.13,39.37
  Bottom 0.305: v42.31,18.27 42.31,21.19 40.64,22.86 v33.02,22.86 | v29.21,25.4 29.21,34.29 v24.13,39.37 | v52.07,13.97 52.07,17.78 v55.88,21.59
  other vias: 63.5,25.4
RX-I  (via drill 0.38)
  Top 0.254: JP11.1B 63.5,49.53
  Top 0.305: U4.30 43.11,15.06 44.2,13.97 48.13,13.97 53.59,19.43 53.59,36.7 63.5,46.61 JP11.1A 63.5,49.53 63.5,50.8 v62.23,50.8 | U1.2 21.72,36.2 v23.37,34.54 24.89,33.02 D3.C
  Bottom 0.305: v62.23,50.8 59.69,48.26 24.13,48.26 21.59,45.72 21.59,40.01 23.37,38.23 v23.37,34.54
SCK  (via drill 0.38, 0.38 pad 0.51)
  Top 0.254: JP2.5B JP2.5A
  Top 0.305: U4.17 v37.62,24.92 36.32,26.21 36.32,27.94 36.83,28.45 36.83,38.86 | J2.3 TP5.P$1 | JP2.5B 28.96,47.24 36.83,39.37 36.83,38.86 | R1.1 36.83,38.86
  Bottom 0.305: v37.62,24.92 37.62,26.06 39.5,27.94 TP5.P$1
  other vias: 63.5,27.94
SHLD  (via drill 0.38)
  other vias: 1.27,43.94 4.19,43.94 1.27,34.8
  pour Bottom: 0,44.45 5.08,44.45 5.08,34.29 0,34.29
  pour Top: 0,44.45 5.08,44.45 5.08,34.29 0,34.29
SS
  Top 0.254: JP2.8A JP2.8B
  Top 0.305: U4.14 40.71,41.84 36.58,45.97 JP2.8B
TX-O  (via drill 0.38)
  Top 0.254: JP11.2A JP11.2B
  Top 0.305: U4.31 43.91,15.27 44.45,14.73 48.01,14.73 52.96,19.68 52.96,37.72 60.96,45.72 JP11.2B | v59.69,50.8 60.96,50.8 JP11.2A | LED5.C 22.86,36.83 22.23,37.47 v21.72,37.47 U1.3
  Bottom 0.305: v59.69,50.8 58.42,49.53 24.13,49.53 20.32,45.72 20.32,39.37 21.72,37.97 v21.72,37.47
USBVCC
  Top 0.508: C15.+ F1.2 7.25,28.06 7.45,27.86 Q1.3 8,26.92 8.76,27.69 C12.1
VCC  (via drill 0.38)
  Top 0.305: v55.88,22.86 55.88,27.94 59.27,31.33 R2.2 63.37,33.78 66.04,31.11 TP1.P$1 J2.2 | R3.2 26.16,27.3 v25.59,27.88 19.34,34.12 10.58,34.12 | R6.2 57.66,13.97 | 57.66,13.97 R13.2 | v57.66,15.24 57.66,13.97 | C18.1 10.58,34.12 | R12.2 v25.78,31.11 | R16.2 v25.78,34.92 | U1.16 8.51,34.92 9.31,34.12 10.58,34.12
  Top 0.508: U4.6 44.52,21.52 44.07,21.97 42.29,21.97 41.91,21.59 | C2.2 U4.18 39.91,22.32 v40.64,21.59 41.91,21.59 | v47.77,19.92 U4.4 42.31,19.92 41.91,20.32 41.91,21.59 | v31.75,21.59 30.48,22.86 27.94,22.86 | I/O.2 27.94,22.86 | R3.2 27.09,25.49 27.94,24.64 27.94,22.86
  Bottom 0.305: v47.77,19.92 52.94,19.92 v55.88,22.86 57.15,22.86 57.66,22.35 v57.66,15.24 | v25.78,34.92 v25.78,31.11 25.78,28.07 v25.59,27.88
  Bottom 0.508: v40.64,21.59 v31.75,21.59
  other vias: 66.04,30.48
VIN  (via drill 0.38)
  Top 0.305: JP10.1 45.72,4.19
  Top 0.762: v29.2,7.1 25.9,7.1 24.76,8.24 C5.+ 17.16,8.24 16,9.4 D1.C 16,21.59 13.72,23.88 IC3.3
  Top 0.813: v41.9,7.1 44.59,7.1 45.72,5.97 45.72,4.19
  Bottom 0.813: v29.2,7.1 v41.9,7.1
VUSB  (via drill 0.38)
  Top 0.381: J1.VBUS 5.08,40.64
  Top 0.508: 5.08,40.64 v5.97,41.53 | F1.1 C10.1 3.43,29.88 v3.43,31.11
  Bottom 0.508: v3.43,31.11 3.43,33.02 3.94,33.53 5.21,33.53 5.71,34.04 5.71,41.27 v5.97,41.53

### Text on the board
Bottom: v10
Measures: Units in inches
tDocu: J. Lindblom, N. Seidle | The Hoff | Based on Arduino by: M. Banzi, D. Cuartielles, / T. Igoe, G. Martino, D. Mellis
214bmp: D:/SmartProjects/Snc/a4_bn_logo2.bmp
